FUNCTION_BLOCK FB_DO_IED_LD1_LEDGGIO7_SPCSO1 EXTENDS FB_AcsiCommonControllableDataClass
VAR_INPUT
	stVal: FB_AcsiBATypeBOOLEAN := (fc:=ACSI_FC_ST, TrgOp:=ACSI_TrgOp_dchg, bLinkResult:=THIS^.AddDataToContainer(ipData:=stVal));
	q: FB_AcsiDATypeQuality := (fc:=ACSI_FC_ST, TrgOp:=ACSI_TrgOp_qchg, bLinkResult:=THIS^.AddDataToContainer(ipData:=q));
	t: FB_AcsiDATypeTimeStamp := (fc:=ACSI_FC_ST, bLinkResult:=THIS^.AddDataToContainer(ipData:=t));
	stSeld: FB_AcsiBATypeBOOLEAN := (fc:=ACSI_FC_ST, TrgOp:=ACSI_TrgOp_dchg, bLinkResult:=THIS^.AddDataToContainer(ipData:=stSeld));
	ctlModel: FB_AcsiDATypeCtlModels := (fc:=ACSI_FC_CF, TrgOp:=ACSI_TrgOp_dchg, eValue:=E_AcsiCtlModels.SBOWithNormalSecurity, bLinkResult:=THIS^.AddDataToContainer(ipData:=ctlModel));
	sboTimeout: FB_AcsiBATypeINT32U := (fc:=ACSI_FC_CF, TrgOp:=ACSI_TrgOp_dchg, nValue:=30000, bLinkResult:=THIS^.AddDataToContainer(ipData:=sboTimeout));
	sboClass: FB_AcsiDATypeSboClasses := (fc:=ACSI_FC_CF, TrgOp:=ACSI_TrgOp_dchg, eValue:=E_AcsiSboClasses.OperateOnce, bLinkResult:=THIS^.AddDataToContainer(ipData:=sboClass));
	operTimeout: FB_AcsiBATypeINT32U := (fc:=ACSI_FC_CF, TrgOp:=ACSI_TrgOp_dchg, nValue:=30000, bLinkResult:=THIS^.AddDataToContainer(ipData:=operTimeout));
	Oper: FB_AcsiCDC_Oper_BOOLEAN := (fc:=ACSI_FC_CO, bLinkResult:=THIS^.AddDataToContainer(ipData:=Oper));
	SBO: FB_AcsiCDC_SBO := (fc:=ACSI_FC_CO, bLinkResult:=THIS^.AddDataToContainer(ipData:=SBO));
	Cancel: FB_AcsiCDC_Cancel_BOOLEAN := (fc:=ACSI_FC_CO, bLinkResult:=THIS^.AddDataToContainer(ipData:=Cancel));
	
	fbControl: FB_SboControl := (ipCtrl:=THIS^.AddServerJob(ipEvent:=fbControl, ipCompletion:=fbControl), eType:=E_AcsiCDCType.SPC, ipBehVal:=fbIED.IEDLD1.LEDGGIO7.Beh.stVal);
END_VAR
VAR
END_VAR

END_FUNCTION_BLOCK
